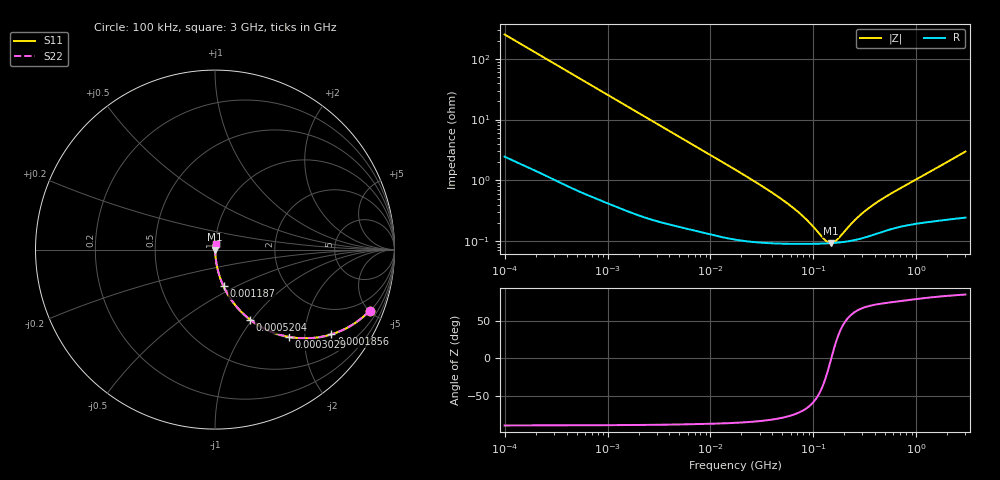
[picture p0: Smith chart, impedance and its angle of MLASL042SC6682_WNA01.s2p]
! MLASL042SC6682_WNA01  S-PARAMETER MODEL  ( Standard Model )
! Model Generated by TAIYO YUDEN Corporation (http://www.ty-top.com)
! Version 1.0
! TAIYO YUDEN Control No. 240524
! Copyright(c) 2024 TAIYO YUDEN CO.,LTD. All Rights Reserved.
! Product Description (link to TY-COMPAS)
! https://ds.yuden.co.jp/TYCOMPAS/or/detail?pn=MLASL042SC6682KWNA01&u=M
! Products Name : Multilayer Ceramic Capacitors
! Characteristics :
!  Capacitance : 6800 [pF] , Rated Voltage : 10 [V] , TCC : X6S
!  Case Size : 0.4 x 0.2 / 0.016 x 0.008 [mm/inch] , Thickness : 0.2 / 0.008 [mm/inch]
!  (Conditions: Temperature = 25 [degC] , DC Bias Voltage = 0 [V])
! External Node Assignments :
!  1  o---| |---o  2
! GND o---------o GND
! Frequency Range : 100kHz  -  3GHz  [ 401 STEP ]
# MHZ S RI R 50
! Freq[MHz].  S11 Real  S11 Imag  S21 Real  S21 Imag  S12 Real  S12 Imag  S22 Real  S22 Imag
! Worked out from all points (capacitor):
!   401 points, 100 kHz to 3 GHz, reference 50 ohm
!   read as one part in series: C = 6.31 nF near 105.3 kHz
!   lowest |Z| = 92.5 mohm at 147.1 MHz (marker M1)
!   series resonance near 149.1 MHz, so ESL is about 180 pH
!   S11 on the Smith chart (normalised r, x): 100 kHz: 1.05, -5.04; 185.6 kHz: 1.03, -2.72; 302.9 kHz: 1.02, -1.68; 520.4 kHz: 1.01, -0.98; 1.187 MHz: 1.01, -0.43; 3 GHz: 1.00, +0.06
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0.1  0.8615 -0.3406  0.1385 0.3406  0.1385 0.3406  0.8615 -0.3406
0.132776  0.7808 -0.4086  0.2192 0.4086  0.2192 0.4086  0.7808 -0.4086
0.185621  0.6483 -0.472  0.3517 0.472  0.3517 0.472  0.6483 -0.472
0.24019  0.5263 -0.4935  0.4737 0.4935  0.4737 0.4935  0.5263 -0.4935
0.302894  0.4135 -0.4864  0.5865 0.4864  0.5865 0.4864  0.4135 -0.4864
0.520403  0.1966 -0.3907  0.8034 0.3907  0.8034 0.3907  0.1966 -0.3907
0.562235  0.1739 -0.3722  0.8261 0.3722  0.8261 0.3722  0.1739 -0.3722
0.786003  0.0992 -0.2914  0.9008 0.2914  0.9008 0.2914  0.0992 -0.2914
1.18716  0.0478 -0.2049  0.9522 0.2049  0.9522 0.2049  0.0478 -0.2049
3.161081  0.00867 -0.0809  0.9913 0.0809  0.9913 0.0809  0.00867 -0.0809
17.7727  0.00126 -0.0146  0.9987 0.0146  0.9987 0.0146  0.00126 -0.0146
52.46276  0.000923 -0.00442  0.9991 0.00442  0.9991 0.00442  0.000923 -0.00442
73.34282  0.000904 -0.00274  0.9991 0.00274  0.9991 0.00274  0.000904 -0.00274
97.38194  0.000902 -0.00156  0.9991 0.00156  0.9991 0.00156  0.000902 -0.00156
129.3002  0.000913 -0.000509  0.9991 0.000509  0.9991 0.000509  0.000913 -0.000509
147.0833  0.000923 -4.91e-05  0.9991 4.91e-05  0.9991 4.91e-05  0.000923 -4.91e-05
158.9065  0.000932 0.000226  0.9991 -0.000226  0.9991 -0.000226  0.000932 0.000226
171.6802  0.000943 0.000502  0.9991 -0.000502  0.9991 -0.000502  0.000943 0.000502
240.0085  0.00102 0.00175  0.999 -0.00175  0.999 -0.00175  0.00102 0.00175
310.5665  0.00114 0.0028  0.9989 -0.0028  0.9989 -0.0028  0.00114 0.0028
547.5153  0.00157 0.00561  0.9984 -0.00561  0.9984 -0.00561  0.00157 0.00561
3000  0.00329 0.0295  0.9967 -0.0295  0.9967 -0.0295  0.00329 0.0295
